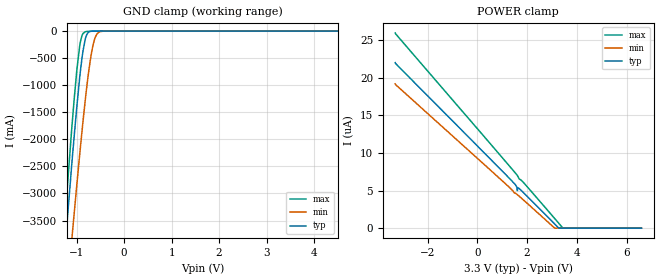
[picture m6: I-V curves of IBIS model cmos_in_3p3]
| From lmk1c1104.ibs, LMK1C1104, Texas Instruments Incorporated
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[Model]   cmos_in_3p3
Model_type   Input
Vinl = 0.99
Vinh = 2.31
|   typ   min   max
C_comp   6.995pF   6.6285pF   7.495pF
[Voltage Range]   3.3   3.135   3.465
[Temperature Range]   25   150   -40
[Power Clamp Reference]   3.3   3.135   3.465
[GND Clamp Reference]   0   0   0
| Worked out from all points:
|   GND clamp passes 1 mA (typ) near -0.65 V on its own axis
[GND Clamp]
|   Voltage   I(typ)   I(min)   I(max)
-3.3V     -25.56A    -22.58A    -30.68A
-1.399V   -5.695A    -6.834A    -5.263A
-1.092V   -2.371A    -3.773A    -1.7A
-1.073V   -2.167A    -3.581A    -1.487A
-993.3mV  -1.385A    -2.826A    -707.2mA
-933.9mV  -856.7mA   -2.278A    -273.7mA
-884.4mV  -488.2mA   -1.837A    -78.77mA
-815.1mV  -140.6mA   -1.259A    -11.82mA
-726mV    -10.83mA   -628.9mA   -3.242mA
-646.8mV  -983.3uA   -234.5mA   -880.4uA
-488.4mV  -15.7uA    -7.205mA   -16.49uA
6.6V      0A         0A         0A
[POWER Clamp]
|   Voltage   I(typ)   I(min)   I(max)
-3.3V     21.99uA    19.17uA    25.95uA
1.432V    6.133uA    4.944uA    7.71uA
1.482V    5.958uA    4.711uA    7.516uA
1.601V    5.407uA    4.479uA    7.034uA
1.61V     4.979uA    4.452uA    6.988uA
1.62V     5.365uA    4.425uA    6.938uA
1.709V    5.186uA    4.17uA     6.475uA
1.907V    4.553uA    3.589uA    5.874uA
3.105V    573.8nA    17.57nA    1.304uA
3.274V    11.08nA    0A         657.3nA
3.442V    0A         0A         10.14nA
6.6V      0A         0A         0A
